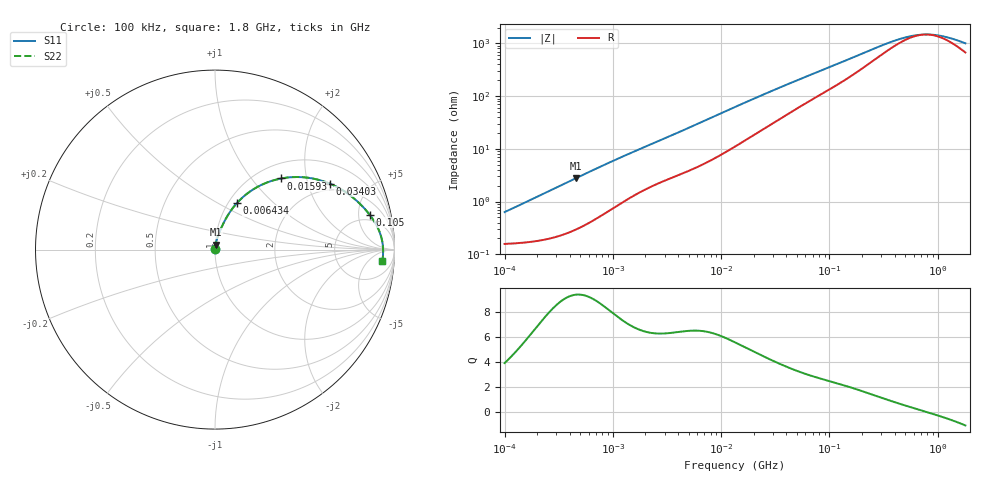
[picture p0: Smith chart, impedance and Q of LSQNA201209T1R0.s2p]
! LSQNA201209T1R0  S-PARAMETER MODEL  ( General Type )
! Model Generated by TAIYO YUDEN Corporation (http://www.ty-top.com)
! Version 2.0
! TAIYO YUDEN Control No. 100810NF25SB-FKC
! Copyright(c) 2007 TAIYO YUDEN CO.,LTD. All Rights Reserved.
! Product Description (link to TY-COMPAS)
! https://ds.yuden.co.jp/TYCOMPAS/or/detail?pn=LSQNA201209T1R0M&u=M
! Products Name : Inductors
! Characteristics :
!  Inductance : 1.0 uH , SRF(min) : 100 MHz , DC Resistance(max) : 0.195 Ohm
!  Rated Current : Saturation :620 mA , Temp Rise : 950 mA (40 degC)
!  Case Size : 2.0 x 1.25 / 0.079 x 0.049 [mm/inch] , Thickness : 0.9 / 0.035 [mm/inch]
!  (Conditions: Temperature = 25 degC , DC Bias Current/Voltage = 0A / 0V)
! External Node Assignments :
!  1  o---GGG---o  2
! GND o---------o GND
! Frequency Range : 0.1MHz  -  1800MHz  [ 402 STEP ]
# MHz S RI R 50
! Freq[MHz].  S11 Real  S11 Imag  S21 Real  S21 Imag  S12 Real  S12 Imag  S22 Real  S22 Imag
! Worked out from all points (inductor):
!   401 points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, 100 kHz to 1.8 GHz, reference 50 ohm
!   read as one part in series: L = 974 nH near 105 kHz
!   highest Q = 9.37 at 456.6 kHz (marker M1), where L = 964 nH
!   self-resonance near 769.8 MHz
!   S11 on the Smith chart (normalised r, x): 100 kHz: 1.00, +0.01; 6.434 MHz: 1.10, +0.62; 15.93 MHz: 1.27, +1.43; 34.03 MHz: 1.72, +2.77; 105 MHz: 3.84, +6.79; 1.8 GHz: 14, -15
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0.1  0.00161 0.0061  0.9984 -0.0061  0.9984 -0.0061  0.00161 0.0061
0.456633  0.0037 0.0275  0.9963 -0.0275  0.9963 -0.0275  0.0037 0.0275
0.516129  0.00428 0.0309  0.9957 -0.0309  0.9957 -0.0309  0.00428 0.0309
1.246616  0.0147 0.0699  0.9853 -0.0699  0.9853 -0.0699  0.0147 0.0699
2.66389  0.0399 0.1315  0.9601 -0.1315  0.9601 -0.1315  0.0399 0.1315
4.347904  0.0736 0.1945  0.9264 -0.1945  0.9264 -0.1945  0.0736 0.1945
6.434145  0.1233 0.2604  0.8767 -0.2604  0.8767 -0.2604  0.1233 0.2604
9.291023  0.1999 0.3268  0.8001 -0.3268  0.8001 -0.3268  0.1999 0.3268
13.41641  0.3093 0.3808  0.6907 -0.3808  0.6907 -0.3808  0.3093 0.3808
15.92588  0.3693 0.3963  0.6307 -0.3963  0.6307 -0.3963  0.3693 0.3963
22.99727  0.5047 0.4019  0.4953 -0.4019  0.4953 -0.4019  0.5047 0.4019
34.03197  0.6384 0.3681  0.3616 -0.3681  0.3616 -0.3681  0.6384 0.3681
47.95365  0.7314 0.3178  0.2686 -0.3178  0.2686 -0.3178  0.7314 0.3178
69.24595  0.8041 0.2584  0.1959 -0.2584  0.1959 -0.2584  0.8041 0.2584
105.0131  0.8609 0.1953  0.1391 -0.1953  0.1391 -0.1953  0.8609 0.1953
184.4683  0.9068 0.1217  0.0932 -0.1217  0.0932 -0.1217  0.9068 0.1217
357.3983  0.9297 0.0559  0.0703 -0.0559  0.0703 -0.0559  0.9297 0.0559
555.4434  0.9351 0.0224  0.0649 -0.0224  0.0649 -0.0224  0.9351 0.0224
675.6865  0.9361 0.00883  0.0639 -0.00883  0.0639 -0.00883  0.9361 0.00883
802.0705  0.9366 -0.00278  0.0634 0.00278  0.0634 0.00278  0.9366 -0.00278
1130.179  0.9363 -0.0267  0.0637 0.0267  0.0637 0.0267  0.9363 -0.0267
1800  0.9328 -0.0646  0.0672 0.0646  0.0672 0.0646  0.9328 -0.0646
